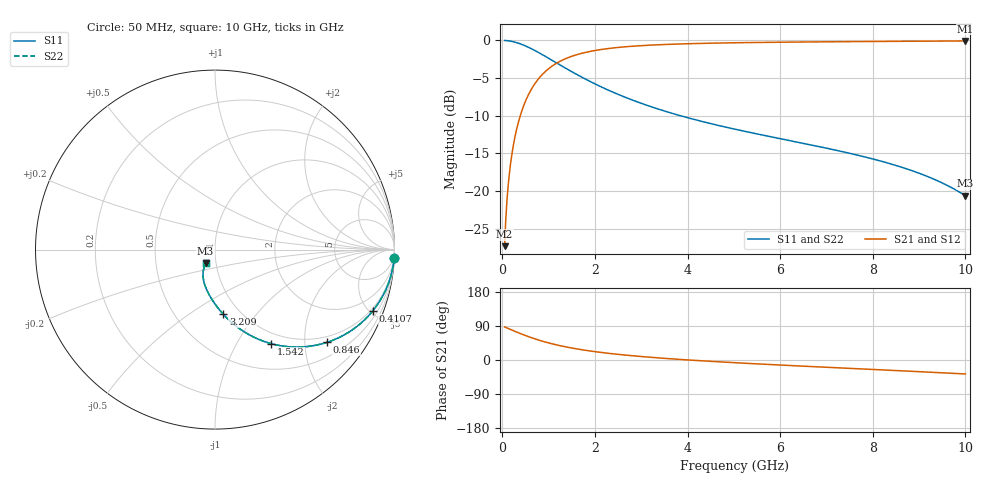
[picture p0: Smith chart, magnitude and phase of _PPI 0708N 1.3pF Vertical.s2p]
! S-Parameter data specifications (vertical orientation):
! Substrate: 40-mil Rogers 3003C, Substrate thickness, H=1.016mm, Dielectric constant, Er=3, Conductor thickness, T_mtl=0.043mm, Loss Tangent, Tand=0.003
! PCB Mounting Pad Footprint: Pad width, PadW=2.54mm , Pad length, PadL=0.51mm , Pad gap, PadG (edge-to-edge)=0.71mm , Reference planes=1.73mm apart
! Created Tue Jan 16 08:42:56 2018
# GHz S MA R 50
! 2 Port Network Data from SP1.SP block
! freq  magS11  angS11  magS21  angS21  magS12  angS12  magS22  angS22
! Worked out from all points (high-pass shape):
!   801 points, 50 MHz to 10 GHz, reference 50 ohm
!   highest |S21| = -0.07 dB at 10 GHz (marker M1); lowest = -27.3 dB at 50 MHz (marker M2)
!   |S21| within 3 dB of the highest: 1.161 GHz to end of sweep
!   lowest |S11| = -20.6 dB at 10 GHz (marker M3), VSWR 1.20, Z = 44.5 - j6.87 ohm
!   |S11| at or under -10 dB: 3.84 GHz to end of sweep
!   |S22| runs from -20.6 to 0.0 dB; largest |S21 - S12| = 0
!   S11 on the Smith chart (normalised r, x): 50 MHz: 1, -43; 410.7 MHz: 0.84, -5.20; 846 MHz: 0.84, -2.53; 1.542 GHz: 0.84, -1.40; 3.209 GHz: 0.83, -0.69; 10 GHz: 0.89, -0.14
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0.05  0.9991 -2.7  0.04291 87.3  0.04291 87.3  0.9991 -2.7
0.074875  0.9979 -4.0  0.06419 86.0  0.06419 86.0  0.9979 -4.0
0.1370625  0.9931 -7.3  0.1169 82.7  0.1169 82.7  0.9931 -7.3
0.1619375  0.9904 -8.6  0.1378 81.4  0.1378 81.4  0.9904 -8.6
0.19925  0.9856 -10.6  0.1687 79.4  0.1687 79.4  0.9856 -10.6
0.2863125  0.971 -15.1  0.2387 74.9  0.2387 74.9  0.971 -15.1
0.4106875  0.9431 -21.2  0.3323 68.7  0.3323 68.7  0.9431 -21.2
0.59725  0.8901 -29.8  0.4554 60.2  0.4554 60.2  0.8901 -29.8
0.846  0.8103 -39.6  0.5855 50.4  0.5855 50.4  0.8103 -39.6
1.19425  0.7017 -50.7  0.7118 39.2  0.7118 39.2  0.7017 -50.7
1.5425  0.6092 -59.3  0.7922 30.7  0.7922 30.7  0.6092 -59.3
1.716625  0.5697 -62.8  0.821 27.1  0.821 27.1  0.5697 -62.8
2.015125  0.5115 -68.1  0.8583 21.8  0.8583 21.8  0.5115 -68.1
2.363375  0.4564 -73.2  0.8886 16.7  0.8886 16.7  0.4564 -73.2
3.209125  0.3628 -82.7  0.9305 7.1  0.9305 7.1  0.3628 -82.7
3.370812  0.3494 -84.3  0.9355 5.5  0.9355 5.5  0.3494 -84.3
4.117063  0.2998 -90.4  0.9524 -0.7  0.9524 -0.7  0.2998 -90.4
5.025  0.2569 -96.8  0.9645 -7.2  0.9645 -7.2  0.2569 -96.8
6.691625  0.2012 -106.8  0.9771 -17.4  0.9771 -17.4  0.2012 -106.8
8.345812  0.1524 -115.9  0.9852 -27.0  0.9852 -27.0  0.1524 -115.9
9.25375  0.1221 -120.8  0.989 -32.3  0.989 -32.3  0.1221 -120.8
10  0.09283 -124.5  0.9916 -36.8  0.9916 -36.8  0.09283 -124.5
